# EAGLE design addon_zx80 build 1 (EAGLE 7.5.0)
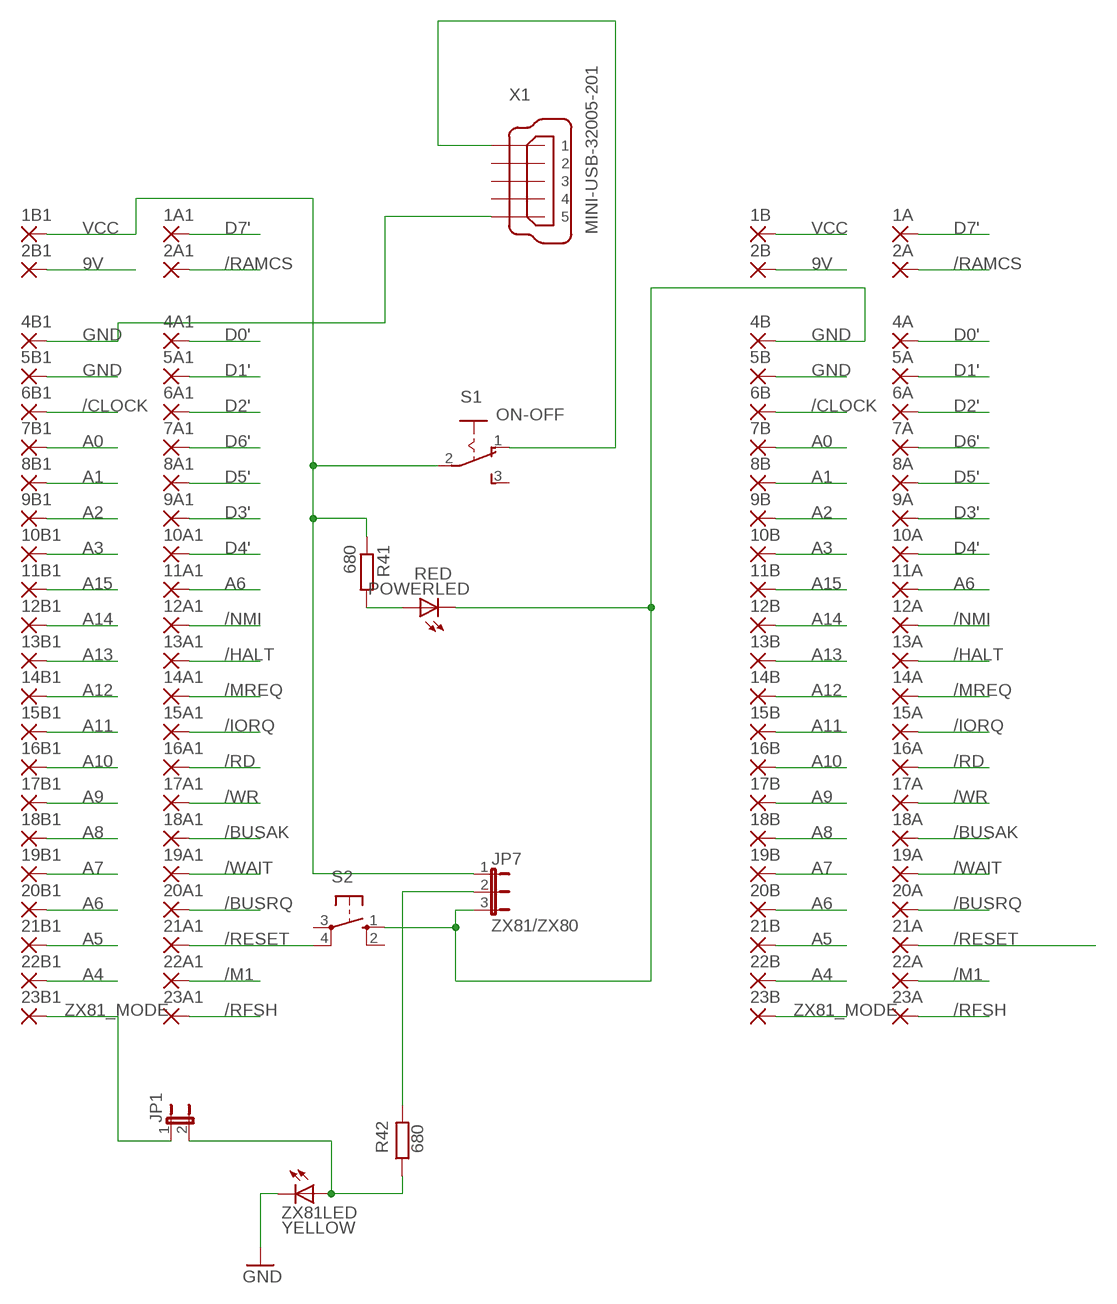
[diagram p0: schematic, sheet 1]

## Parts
1A  SMD2EDGEPIN_SMALL  [EDGEPIN_SMALL]
1A1  SMD2EDGEPIN  [EDGEPIN]
1B  SMD2EDGEPIN_SMALL  [EDGEPIN_SMALL]
1B1  SMD2EDGEPIN  [EDGEPIN]
2A  SMD2EDGEPIN_SMALL  [EDGEPIN_SMALL]
2A1  SMD2EDGEPIN  [EDGEPIN]
2B  SMD2EDGEPIN_SMALL  [EDGEPIN_SMALL]
2B1  SMD2EDGEPIN  [EDGEPIN]
4A  SMD2EDGEPIN_SMALL  [EDGEPIN_SMALL]
4A1  SMD2EDGEPIN  [EDGEPIN]
4B  SMD2EDGEPIN_SMALL  [EDGEPIN_SMALL]
4B1  SMD2EDGEPIN  [EDGEPIN]
5A  SMD2EDGEPIN_SMALL  [EDGEPIN_SMALL]
5A1  SMD2EDGEPIN  [EDGEPIN]
5B  SMD2EDGEPIN_SMALL  [EDGEPIN_SMALL]
5B1  SMD2EDGEPIN  [EDGEPIN]
6A  SMD2EDGEPIN_SMALL  [EDGEPIN_SMALL]
6A1  SMD2EDGEPIN  [EDGEPIN]
6B  SMD2EDGEPIN_SMALL  [EDGEPIN_SMALL]
6B1  SMD2EDGEPIN  [EDGEPIN]
7A  SMD2EDGEPIN_SMALL  [EDGEPIN_SMALL]
7A1  SMD2EDGEPIN  [EDGEPIN]
7B  SMD2EDGEPIN_SMALL  [EDGEPIN_SMALL]
7B1  SMD2EDGEPIN  [EDGEPIN]
8A  SMD2EDGEPIN_SMALL  [EDGEPIN_SMALL]
8A1  SMD2EDGEPIN  [EDGEPIN]
8B  SMD2EDGEPIN_SMALL  [EDGEPIN_SMALL]
8B1  SMD2EDGEPIN  [EDGEPIN]
9A  SMD2EDGEPIN_SMALL  [EDGEPIN_SMALL]
9A1  SMD2EDGEPIN  [EDGEPIN]
9B  SMD2EDGEPIN_SMALL  [EDGEPIN_SMALL]
9B1  SMD2EDGEPIN  [EDGEPIN]
10A  SMD2EDGEPIN_SMALL  [EDGEPIN_SMALL]
10A1  SMD2EDGEPIN  [EDGEPIN]
10B  SMD2EDGEPIN_SMALL  [EDGEPIN_SMALL]
10B1  SMD2EDGEPIN  [EDGEPIN]
11A  SMD2EDGEPIN_SMALL  [EDGEPIN_SMALL]
11A1  SMD2EDGEPIN  [EDGEPIN]
11B  SMD2EDGEPIN_SMALL  [EDGEPIN_SMALL]
11B1  SMD2EDGEPIN  [EDGEPIN]
12A  SMD2EDGEPIN_SMALL  [EDGEPIN_SMALL]
12A1  SMD2EDGEPIN  [EDGEPIN]
12B  SMD2EDGEPIN_SMALL  [EDGEPIN_SMALL]
12B1  SMD2EDGEPIN  [EDGEPIN]
13A  SMD2EDGEPIN_SMALL  [EDGEPIN_SMALL]
13A1  SMD2EDGEPIN  [EDGEPIN]
13B  SMD2EDGEPIN_SMALL  [EDGEPIN_SMALL]
13B1  SMD2EDGEPIN  [EDGEPIN]
14A  SMD2EDGEPIN_SMALL  [EDGEPIN_SMALL]
14A1  SMD2EDGEPIN  [EDGEPIN]
14B  SMD2EDGEPIN_SMALL  [EDGEPIN_SMALL]
14B1  SMD2EDGEPIN  [EDGEPIN]
15A  SMD2EDGEPIN_SMALL  [EDGEPIN_SMALL]
15A1  SMD2EDGEPIN  [EDGEPIN]
15B  SMD2EDGEPIN_SMALL  [EDGEPIN_SMALL]
15B1  SMD2EDGEPIN  [EDGEPIN]
16A  SMD2EDGEPIN_SMALL  [EDGEPIN_SMALL]
16A1  SMD2EDGEPIN  [EDGEPIN]
16B  SMD2EDGEPIN_SMALL  [EDGEPIN_SMALL]
16B1  SMD2EDGEPIN  [EDGEPIN]
17A  SMD2EDGEPIN_SMALL  [EDGEPIN_SMALL]
17A1  SMD2EDGEPIN  [EDGEPIN]
17B  SMD2EDGEPIN_SMALL  [EDGEPIN_SMALL]
17B1  SMD2EDGEPIN  [EDGEPIN]
18A  SMD2EDGEPIN_SMALL  [EDGEPIN_SMALL]
18A1  SMD2EDGEPIN  [EDGEPIN]
18B  SMD2EDGEPIN_SMALL  [EDGEPIN_SMALL]
18B1  SMD2EDGEPIN  [EDGEPIN]
19A  SMD2EDGEPIN_SMALL  [EDGEPIN_SMALL]
19A1  SMD2EDGEPIN  [EDGEPIN]
19B  SMD2EDGEPIN_SMALL  [EDGEPIN_SMALL]
19B1  SMD2EDGEPIN  [EDGEPIN]
20A  SMD2EDGEPIN_SMALL  [EDGEPIN_SMALL]
20A1  SMD2EDGEPIN  [EDGEPIN]
20B  SMD2EDGEPIN_SMALL  [EDGEPIN_SMALL]
20B1  SMD2EDGEPIN  [EDGEPIN]
21A  SMD2EDGEPIN_SMALL  [EDGEPIN_SMALL]
21A1  SMD2EDGEPIN  [EDGEPIN]
21B  SMD2EDGEPIN_SMALL  [EDGEPIN_SMALL]
21B1  SMD2EDGEPIN  [EDGEPIN]
22A  SMD2EDGEPIN_SMALL  [EDGEPIN_SMALL]
22A1  SMD2EDGEPIN  [EDGEPIN]
22B  SMD2EDGEPIN_SMALL  [EDGEPIN_SMALL]
22B1  SMD2EDGEPIN  [EDGEPIN]
23A  SMD2EDGEPIN_SMALL  [EDGEPIN_SMALL]
23A1  SMD2EDGEPIN  [EDGEPIN]
23B  SMD2EDGEPIN_SMALL  [EDGEPIN_SMALL]
23B1  SMD2EDGEPIN  [EDGEPIN]
JP1  JP1E  [JP1]
JP7  ZX81/ZX80  JP2E  [JP2]
POWERLED  RED  LED3MM  [LED3MM]
R41  680  R-EU_0204/7  [0204/7]
R42  680  R-EU_0204/7  [0204/7]
S1  ON-OFF  255SB  [255SB]
S2  10-XX  [B3F-10XX]
X1  MINI-USB-32005-201  [32005-201]
ZX81LED  YELLOW  LED3MM  [LED3MM]

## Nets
9V: 2B1.1(P) 2B.1(P)
/BUSAK: 18A1.1(P) 18A.1(P)
/BUSRQ: 20A1.1(P) 20A.1(P)
/CLOCK: 6B1.1(P) 6B.1(P)
/HALT: 13A1.1(P) 13A.1(P)
/IORQ: 15A1.1(P) 15A.1(P)
/M1: 22A1.1(P) 22A.1(P)
/MREQ: 14A1.1(P) 14A.1(P)
/NMI: 12A1.1(P) 12A.1(P)
/RAMCS: 2A1.1(P) 2A.1(P)
/RD: 16A1.1(P) 16A.1(P)
/RESET: 21A1.1(P) 21A.1(P) S2.4(P1)
/RFSH: 23A1.1(P) 23A.1(P)
/WAIT: 19A1.1(P) 19A.1(P)
/WR: 17A1.1(P) 17A.1(P)
A0: 7B1.1(P) 7B.1(P)
A1: 8B1.1(P) 8B.1(P)
A2: 9B1.1(P) 9B.1(P)
A3: 10B1.1(P) 10B.1(P)
A4: 22B1.1(P) 22B.1(P)
A5: 21B1.1(P) 21B.1(P)
A6: 11A1.1(P) 11A.1(P) 20B1.1(P) 20B.1(P)
A7: 19B1.1(P) 19B.1(P)
A8: 18B1.1(P) 18B.1(P)
A9: 17B1.1(P) 17B.1(P)
A10: 16B1.1(P) 16B.1(P)
A11: 15B1.1(P) 15B.1(P)
A12: 14B1.1(P) 14B.1(P)
A13: 13B1.1(P) 13B.1(P)
A14: 12B1.1(P) 12B.1(P)
A15: 11B1.1(P) 11B.1(P)
D0': 4A1.1(P) 4A.1(P)
D1': 5A1.1(P) 5A.1(P)
D2': 6A1.1(P) 6A.1(P)
D3': 9A1.1(P) 9A.1(P)
D4': 10A1.1(P) 10A.1(P)
D5': 8A1.1(P) 8A.1(P)
D6': 7A1.1(P) 7A.1(P)
D7': 1A1.1(P) 1A.1(P)
GND: 4B1.1(P) 4B.1(P) 5B1.1(P) 5B.1(P) JP7.3 POWERLED.K(C) S2.1(S) X1.5 ZX81LED.K(C)
N$1: S1.1(O) X1.1
N$8: POWERLED.A R41.2
VCC [VCC]: 1B1.1(P) 1B.1(P) JP7.1 R41.1 S1.2(P)
XXXX: JP7.2 R42.2
ZX81_MODE: 23B1.1(P) 23B.1(P) JP1.1
ZX81_MODE': JP1.2 R42.1 ZX81LED.A
Unconnected: S1.3(S) S2.2(S1) S2.3(P) X1.2 X1.3 X1.4

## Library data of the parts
1A 1A1 1B 1B1 2A 2A1 2B 2B1 4A 4A1 4B 4B1 5A 5A1 5B 5B1 6A 6A1 6B 6B1 7A 7A1 7B 7B1 8A 8A1 8B 8B1 9A 9A1 9B 9B1 10A 10A1 10B 10B1 11A 11A1 11B 11B1 12A 12A1 12B 12B1 13A 13A1 13B 13B1 14A 14A1 14B 14B1 15A 15A1 15B 15B1 16A 16A1 16B 16B1 17A 17A1 17B 17B1 18A 18A1 18B 18B1 19A 19A1 19B 19B1 20A 20A1 20B 20B1 21A 21A1 21B 21B1 22A 22A1 22B 22B1 23A 23A1 23B 23B1 = wirepad:SMD2: SMD PAD
JP1 = jumper:JP1E: JUMPER
JP7 = jumper:JP2E: JUMPER
POWERLED ZX81LED = led:LED: LED
R41 R42 = resistor:R-EU_: RESISTOR, European symbol
S1 = switch:255SB: SLIDING SWITCH Distributor Buerklin, 11G810
S2 = switch-omron:10-XX: OMRON SWITCH; MPN: B3F-1000; OC_FARNELL: 176432; OC_NEWARK: 36M3542
X1 = con-cypressindustries:MINI-USB-: MINI USB-B Conector Source: www.cypressindustries.com; OC_FARNELL: unknown; OC_NEWARK: unknown

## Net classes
1 VCC: width 0.5 mm

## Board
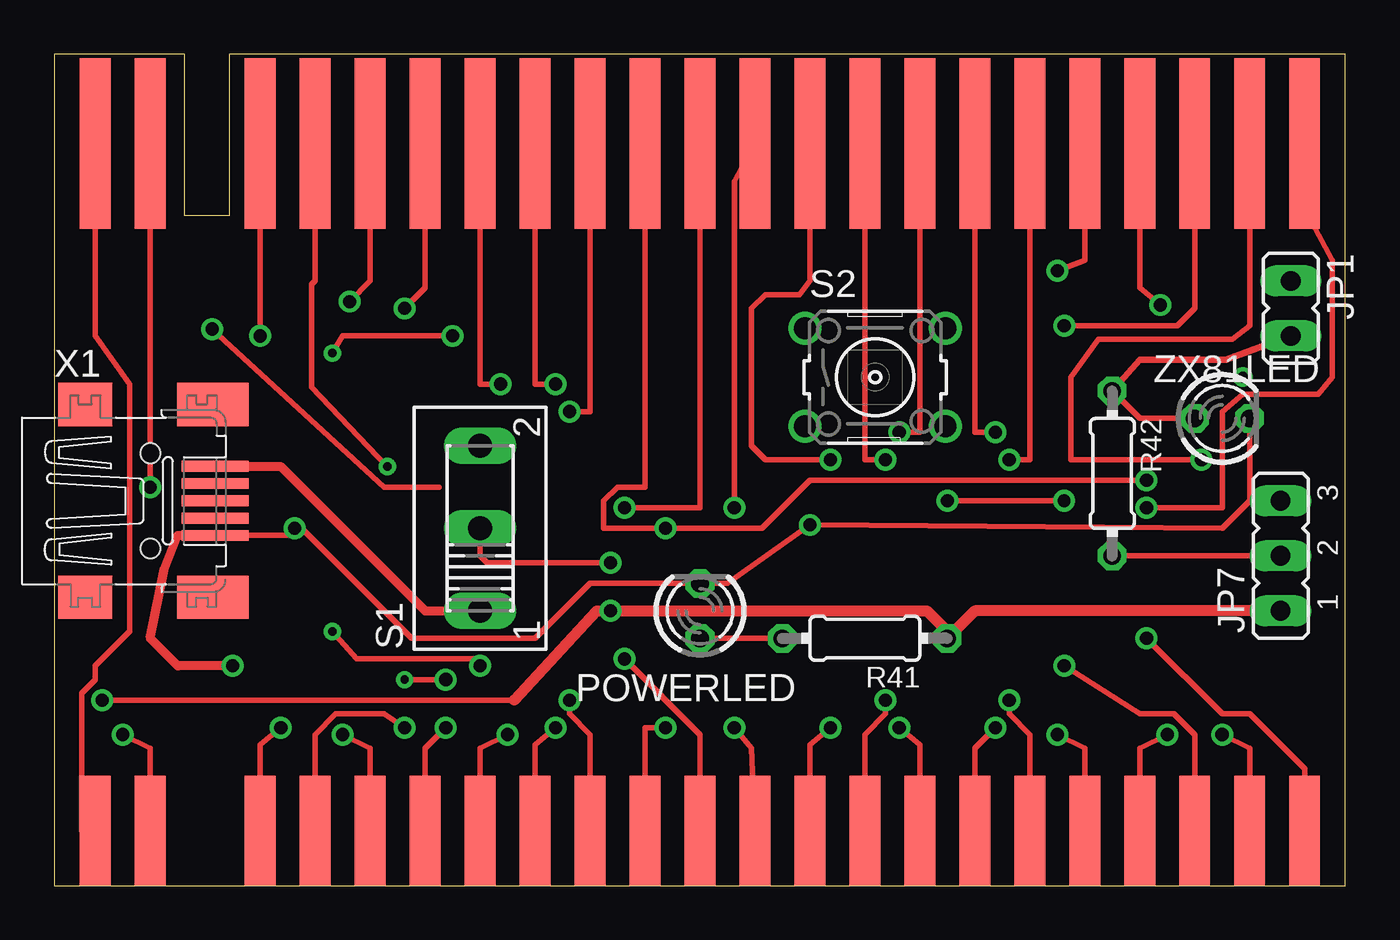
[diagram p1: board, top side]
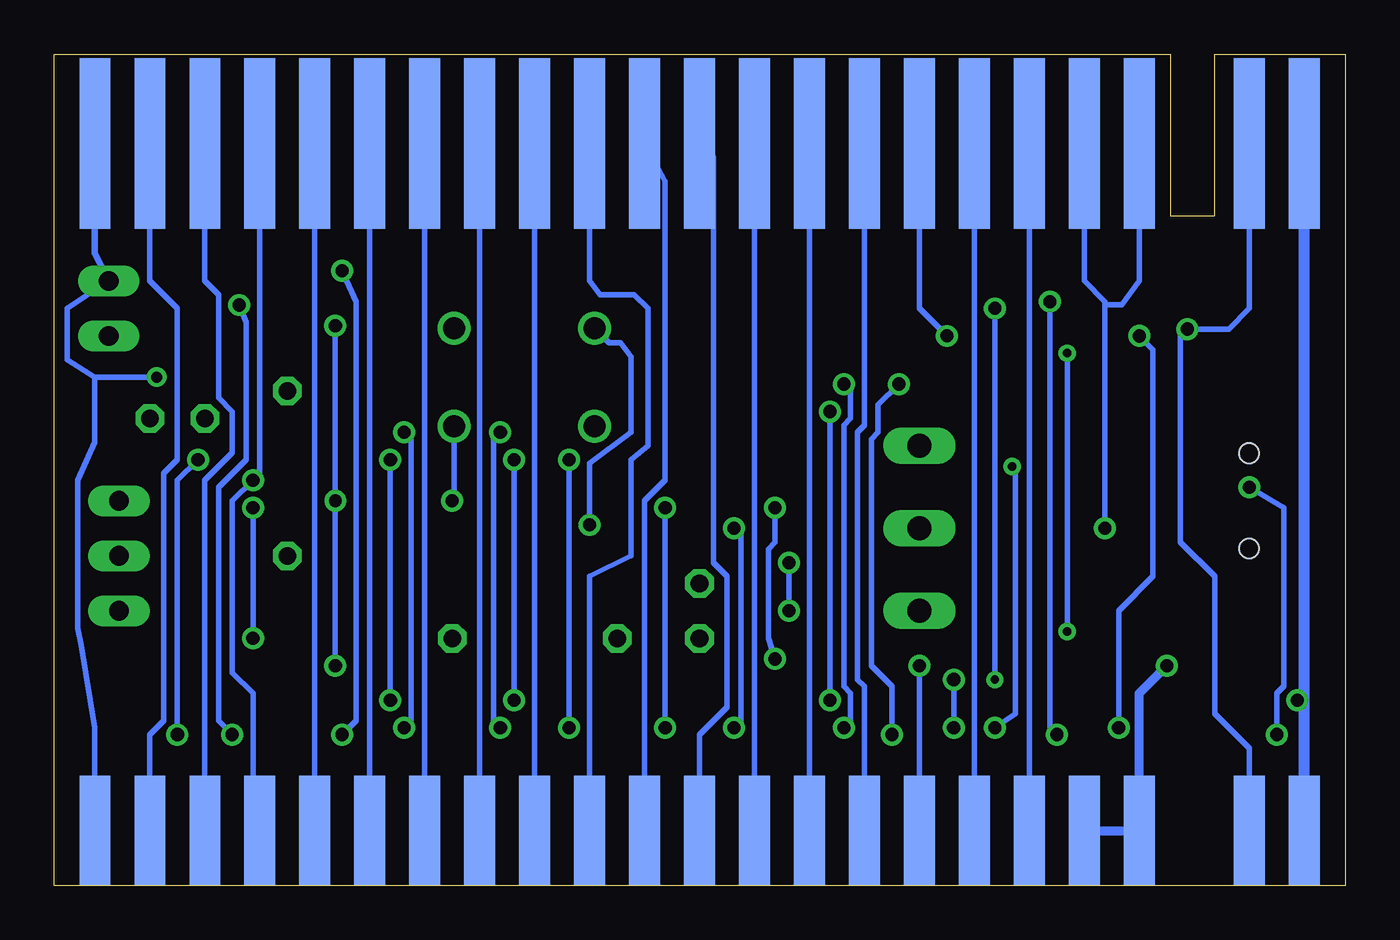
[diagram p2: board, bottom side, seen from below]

Size 59.67 x 38.42 mm. Coordinates in mm from the lower left corner, seen from the top.
Outline: 0,0 59.67,0 59.67,38.41 8.1,38.42 8.1,30.96 6.03,30.96 6.03,38.42 5.56,38.42 0,38.41 0,0
Copper layers (1*16): Top 0.035mm / dielectric 1.5mm / Bottom 0.035mm
Design rules "default": minimum track width 10mil, minimum drill 24mil, track to track 8mil, track to pad 8mil, pad to pad 8mil, via to via 8mil, smd to smd 8mil, copper to edge 40mil, drill to drill 8mil, minimum pad ring 10mil, minimum via ring 8mil, stop-mask expansion 4mil, vias tented up to drill 0mil, thermal gap 10mil

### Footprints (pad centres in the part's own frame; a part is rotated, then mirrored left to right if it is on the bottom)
EDGEPIN_SMALL = smd 1.422 x 5.08: 1 0,0
EDGEPIN = smd 1.422 x 7.874: 1 0,0
JP1 = drill 0.914 long: 1 0,-1.27; 2 0,1.27
JP2 = drill 0.914 long: 1 -2.54,0; 2 0,0; 3 2.54,0
LED3MM = drill 0.813 octagon: A -1.27,0; K 1.27,0
0204/7 = drill 0.813 octagon: 1 -3.81,0; 2 3.81,0
255SB = drill 1.118 long: 1 -3.81,0; 2 0,0; 3 3.81,0
B3F-10XX = drill 1.016: 1 -3.251,2.261; 2 3.251,2.261; 3 -3.251,-2.261; 4 3.251,-2.261
32005-201 = smd 3.1 x 0.5: 1 3,1.6; 2 3,0.8; 3 3,0; 4 3,-0.8; 5 3,-1.6 | smd 2.5 x 2: M1 -3,-4.45; M2 -3,4.45 | smd 3.3 x 2: M3 2.9,4.45; M4 2.9,-4.45 | hole 0.9: 0,2.2; 0,-2.2

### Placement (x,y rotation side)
1A  1.91,2.54 0 top
1A1  1.91,34.29 0 top
1B  1.91,2.54 180 bottom
1B1  1.91,34.29 180 bottom
2A  4.45,2.54 0 top
2A1  4.45,34.29 0 top
2B  4.45,2.54 180 bottom
2B1  4.45,34.29 180 bottom
4A  9.53,2.54 0 top
4A1  9.53,34.29 0 top
4B  9.53,2.54 180 bottom
4B1  9.53,34.29 180 bottom
5A  12.06,2.54 0 top
5A1  12.06,34.29 0 top
5B  12.06,2.54 180 bottom
5B1  12.06,34.29 180 bottom
6A  14.61,2.54 0 top
6A1  14.61,34.29 0 top
6B  14.61,2.54 180 bottom
6B1  14.61,34.29 180 bottom
7A  17.15,2.54 0 top
7A1  17.15,34.29 0 top
7B  17.15,2.54 180 bottom
7B1  17.15,34.29 180 bottom
8A  19.69,2.54 0 top
8A1  19.69,34.29 0 top
8B  19.69,2.54 180 bottom
8B1  19.69,34.29 180 bottom
9A  22.23,2.54 0 top
9A1  22.23,34.29 0 top
9B  22.23,2.54 180 bottom
9B1  22.23,34.29 180 bottom
10A  24.77,2.54 0 top
10A1  24.77,34.29 0 top
10B  24.77,2.54 180 bottom
10B1  24.77,34.29 180 bottom
11A  27.31,2.54 0 top
11A1  27.31,34.29 0 top
11B  27.31,2.54 180 bottom
11B1  27.31,34.29 180 bottom
12A  29.85,2.54 0 top
12A1  29.85,34.29 0 top
12B  29.85,2.54 180 bottom
12B1  29.85,34.29 180 bottom
13A  32.38,2.54 0 top
13A1  32.38,34.29 0 top
13B  32.38,2.54 180 bottom
13B1  32.38,34.29 180 bottom
14A  34.92,2.54 0 top
14A1  34.92,34.29 0 top
14B  34.92,2.54 180 bottom
14B1  34.92,34.29 180 bottom
15A  37.46,2.54 0 top
15A1  37.46,34.29 0 top
15B  37.46,2.54 180 bottom
15B1  37.46,34.29 180 bottom
16A  40,2.54 0 top
16A1  40,34.29 0 top
16B  40,2.54 180 bottom
16B1  40,34.29 180 bottom
17A  42.54,2.54 0 top
17A1  42.54,34.29 0 top
17B  42.54,2.54 180 bottom
17B1  42.54,34.29 180 bottom
18A  45.09,2.54 0 top
18A1  45.09,34.29 0 top
18B  45.09,2.54 180 bottom
18B1  45.09,34.29 180 bottom
19A  47.62,2.54 0 top
19A1  47.62,34.29 0 top
19B  47.62,2.54 180 bottom
19B1  47.62,34.29 180 bottom
20A  50.16,2.54 0 top
20A1  50.16,34.29 0 top
20B  50.16,2.54 180 bottom
20B1  50.16,34.29 180 bottom
21A  52.7,2.54 0 top
21A1  52.7,34.29 0 top
21B  52.7,2.54 180 bottom
21B1  52.7,34.29 180 bottom
22A  55.24,2.54 0 top
22A1  55.24,34.29 0 top
22B  55.24,2.54 180 bottom
22B1  55.24,34.29 180 bottom
23A  57.78,2.54 0 top
23A1  57.78,34.29 0 top
23B  57.78,2.54 180 bottom
23B1  57.78,34.29 180 bottom
JP1  57.15,26.67 180 top
JP7  56.67,15.24 90 top
POWERLED  29.85,12.7 90 top
R41  37.46,11.43 180 top
R42  48.89,19.05 270 top
S1  19.69,16.51 90 top
S2  37.94,23.5 0 top
X1  4.45,17.78 0 top
ZX81LED  53.98,21.59 0 top

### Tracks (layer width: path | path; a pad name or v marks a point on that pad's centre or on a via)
9V  (via drill 0.61)
  Top 0.254: 17.78,18.41 15.24,18.41 v7.3,25.72
  Bottom 0.254: 2B1.1 4.45,26.67 5.4,25.72 v7.3,25.72 7.62,25.4 7.62,15.88 6.03,14.29 6.03,7.94 4.45,6.35 2B.1
/BUSAK  (via drill 0.61)
  Top 0.254: 18A1.1 45.09,19.68 v44.13,19.68 | v44.13,8.57 44.13,7.94 45.09,6.99 18A.1
  Bottom 0.254: v44.13,8.57 v44.13,19.68
/BUSRQ  (via drill 0.61)
  Top 0.254: 20A1.1 50.16,27.62 v51.12,26.83 | v51.43,6.99 50.16,6.35 20A.1
  Bottom 0.254: v51.12,26.83 50.8,26.04 50.8,19.68 52.07,18.41 52.07,7.62 v51.43,6.99
/CLOCK
  Bottom 0.254: 6B.1 6B1.1
/HALT  (via drill 0.61)
  Top 0.254: 13A1.1 31.43,32.54 v31.43,17.46 | v31.43,7.3 32.23,6.35 13A.1
  Bottom 0.254: v31.43,7.3 v31.43,17.46
/IORQ  (via drill 0.61)
  Top 0.254: 15A1.1 37.46,19.68 v38.42,19.68 | v38.42,8.57 38.42,7.94 37.46,6.99 15A.1
  Bottom 0.254: v38.42,8.57 v38.42,19.68
/M1  (via drill 0.61)
  Top 0.254: 22A1.1 55.24,25.88 54.45,25.24 48.26,25.24 46.99,23.5 46.99,19.68 v53.02,19.68 | v53.98,6.99 55.24,6.35 22A.1
  Bottom 0.254: v53.02,19.68 53.98,18.73 v53.98,6.99
/MREQ  (via drill 0.61)
  Top 0.254: 14A1.1 34.92,27.94 34.45,27.3 32.86,27.3 32.23,26.67 32.23,20.32 32.86,19.68 v35.88,19.68 | v35.88,7.3 34.92,6.51 14A.1
  Bottom 0.254: v35.88,7.3 v35.88,19.68
/NMI  (via drill 0.61)
  Top 0.254: 12A1.1 29.85,17.46 v26.35,17.46 | v26.35,10.48 29.85,6.99 12A.1
  Bottom 0.254: v26.35,10.48 26.67,11.43 26.67,15.56 26.35,15.88 v26.35,17.46
/RAMCS  (via drill 0.61)
  Top 0.254: v4.45,18.41 2A1.1 | v3.17,6.99 4.45,6.35 2A.1
  Bottom 0.254: v4.45,18.41 2.86,17.46 2.86,9.21 3.17,8.89 v3.17,6.99
/RD  (via drill 0.61)
  Top 0.254: 16A1.1 40,20.95 v39.05,20.95 | v39.05,7.3 40,6.51 16A.1
  Bottom 0.254: v39.05,20.95 39.37,20.64 39.37,7.62 v39.05,7.3
/RESET  (via drill 0.6, 0.61)
  Top 0.254: 21A1.1 52.7,26.67 51.91,25.88 v46.67,25.88 | v46.67,10.16 50.16,7.94 51.75,7.94 52.7,6.99 21A.1 | v41.27,17.78 v46.67,17.78
  Bottom 0.254: S2.4 41.19,17.86 v41.27,17.78 | v46.67,10.16 v46.67,17.78 v46.67,25.88
/RFSH  (via drill 0.61)
  Top 0.254: 23A1.1 57.94,30.96 59.05,28.89 59.05,23.5 58.42,22.7 54.93,22.7 53.98,21.91 53.98,17.46 v50.48,17.46 | v50.48,11.43 53.98,7.94 55.24,7.94 57.78,5.4 23A.1
  Bottom 0.254: v50.48,11.43 v50.48,17.46
/WAIT  (via drill 0.61)
  Top 0.254: 19A1.1 47.62,28.89 v46.35,28.42 | v46.35,6.99 47.62,6.35 19A.1
  Bottom 0.254: v46.35,28.42 45.72,26.99 45.72,7.62 v46.35,6.99
/WR  (via drill 0.61)
  Top 0.254: 17A1.1 42.54,20.95 v43.5,20.95 | v43.5,7.3 42.54,6.35 17A.1
  Bottom 0.254: v43.5,20.95 43.18,20.64 43.18,7.62 v43.5,7.3
A0
  Bottom 0.254: 7B.1 7B1.1
A1  (via drill 0.38, 0.6)
  Top 0.254: v19.69,10.16 19.37,10.48 13.97,10.48 v12.86,11.75 | v12.86,24.61 13.33,25.4 v18.42,25.4
  Bottom 0.254: 8B.1 v19.69,10.16 | v12.86,11.75 v12.86,24.61 | v18.42,25.4 19.69,26.67 8B1.1
A2
  Bottom 0.254: 9B1.1 22.23,21.27 22.54,20.95 22.54,9.53 22.23,9.21 9B.1
A3
  Bottom 0.254: 10B.1 10B1.1
A4
  Bottom 0.254: 22B1.1 55.24,27.94 53.98,26.67 53.98,19.68 54.61,19.05 54.61,7.62 55.24,6.99 22B.1
A5
  Bottom 0.254: 21B1.1 52.7,27.94 52.07,27.3 52.07,22.54 51.43,21.91 51.43,20 52.7,18.73 21B.1
A6  (via drill 0.61)
  Top 0.254: 11A1.1 27.31,18.41 26.04,18.41 25.4,17.78 25.4,16.51 v28.26,16.51 32.7,16.51 34.92,18.73 v50.48,18.73 | 11A.1 27.31,7.3 v28.26,7.3
  Bottom 0.254: 20B1.1 50.16,19.05 v50.48,18.73 51.43,17.78 51.43,9.84 50.48,8.89 50.48,2.86 20B.1 | v28.26,7.3 27.94,7.62 27.94,16.19 v28.26,16.51
A7
  Bottom 0.254: 19B.1 19B1.1
A8
  Bottom 0.254: 18B.1 18B1.1
A9
  Bottom 0.254: 17B.1 17B1.1
A10
  Bottom 0.254: 16B.1 16B1.1
A11
  Bottom 0.254: 15B.1 15B1.1
A12
  Bottom 0.254: 14B.1 34.92,14.29 33.02,15.24 33.02,19.68 32.23,20.32 32.23,26.67 32.86,27.3 34.45,27.3 34.92,27.94 14B1.1
A13
  Bottom 0.254: 13B.1 32.38,17.78 31.43,18.73 31.43,32.54 13B1.1
A14
  Bottom 0.254: 12B1.1 29.21,33.66 29.21,14.92 28.58,14.29 28.58,8.26 29.85,6.99 12B.1
A15
  Bottom 0.254: 11B.1 11B1.1
D0'  (via drill 0.61)
  Top 0.254: v9.53,25.4 4A1.1 | v10.48,7.3 9.53,6.51 4A.1
  Bottom 0.254: v9.53,25.4 8.89,24.77 8.89,14.29 10.48,12.7 v10.48,7.3
D1'  (via drill 0.38, 0.61)
  Top 0.254: v15.4,19.37 11.91,23.02 11.91,27.78 12.06,27.94 5A1.1 | v16.19,7.3 15.24,7.94 13.02,7.94 12.06,6.99 5A.1
  Bottom 0.254: v15.4,19.37 15.24,19.05 15.24,7.94 v16.19,7.3
D2'  (via drill 0.6, 0.61)
  Top 0.254: v13.33,6.99 14.61,6.35 6A.1 | v13.65,26.99 14.61,27.94 6A1.1
  Bottom 0.254: v13.33,6.99 13.65,7.3 v13.65,26.99
D3'  (via drill 0.61)
  Top 0.254: 9A1.1 22.23,23.18 v23.18,23.18 | v23.18,7.3 22.23,6.51 9A.1
  Bottom 0.254: v23.18,23.18 22.86,22.86 22.86,21.59 23.18,21.27 23.18,9.21 22.86,8.89 22.86,7.62 v23.18,7.3
D4'  (via drill 0.61)
  Top 0.254: 10A1.1 24.77,21.91 v23.81,21.91 | v23.81,8.57 23.81,7.94 24.77,6.99 10A.1
  Bottom 0.254: v23.81,8.57 v23.81,21.91
D5'  (via drill 0.61)
  Top 0.254: 8A1.1 19.69,23.18 v20.64,23.18 | v20.96,6.99 19.69,6.35 8A.1
  Bottom 0.254: v20.64,23.18 21.59,22.23 21.59,20.95 21.91,20.64 21.91,10.16 20.96,9.21 v20.96,6.99
D6'  (via drill 0.38, 0.6, 0.61)
  Top 0.254: v18.1,9.53 v16.19,9.53 | v18.1,7.3 17.15,6.35 7A.1 | v16.19,26.67 17.15,27.62 7A1.1
  Bottom 0.254: v18.1,7.3 v18.1,9.53 | v16.19,9.53 v16.19,26.67
D7'
  Top 0.254: 1A1.1 1.91,25.4 3.49,23.18 3.49,11.75 1.91,10.16 1.91,9.53 1.27,8.89 1.27,2.54 1A.1
GND  (via drill 0.6)
  Top 0.254: 55.24,17.78 ZX81LED.K | JP7.3 55.24,17.78 | 55.24,17.78 53.98,16.51 v34.92,16.67 31.12,13.97 POWERLED.K 24.77,13.97 22.23,11.43 16.51,11.43 11.43,16.51 v11.11,16.51 10.79,16.19 7.46,16.19 X1.5
  Top 0.406: v8.26,10.16 5.71,10.16 4.45,11.43 5.08,14.61 5.71,16.19 7.43,16.19 X1.5
  Bottom 0.254: 5B1.1 12.06,27.94 11.11,26.99 11.11,26.83 | 11.11,26.83 10.32,26.83 9.53,27.94 4B1.1 | v11.11,16.51 11.11,26.83 | v34.92,16.67 34.92,19.53 33.02,20.95 33.02,24.45 33.5,25.08 34.02,25.08 S2.1
  Bottom 0.406: 5B.1 4B.1 9.53,8.89 v8.26,10.16
N$1
  Top 0.406: X1.1 10.46,19.38 17.15,12.7 S1.1
N$8
  Top 0.254: R41.2 POWERLED.A
VCC  (via drill 0.6, 0.61)
  Top 0.254: v2.22,8.57 21.27,8.57 | v25.72,14.92 20,14.92 19.69,15.24 S1.2
  Top 0.5: JP7.1 42.54,12.7 R41.1 41.27,11.75 40.32,12.7 v25.72,12.7 25.08,12.7 21.27,8.57
  Bottom 0.254: v25.72,12.7 v25.72,14.92
  Bottom 0.5: 1B.1 1.91,8.57 | 1.91,8.57 1B1.1 | 1.91,8.57 v2.22,8.57
XXXX
  Top 0.254: JP7.2 R42.2
ZX81_MODE  (via drill 0.5)
  Bottom 0.254: 57.78,23.5 57.78,20.48 58.58,18.73 58.58,11.91 58.42,11.11 57.78,7.3 23B.1 | v54.93,23.5 57.78,23.5 | JP1.1 59.05,26.67 59.05,24.29 57.78,23.5
  Bottom 0.305: JP1.1 57.78,29.21 23B1.1
ZX81_MODE'
  Top 0.254: R42.1 50.16,21.59 ZX81LED.A
  Top 0.305: R42.1 50.16,24.29 54.13,24.29 JP1.2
